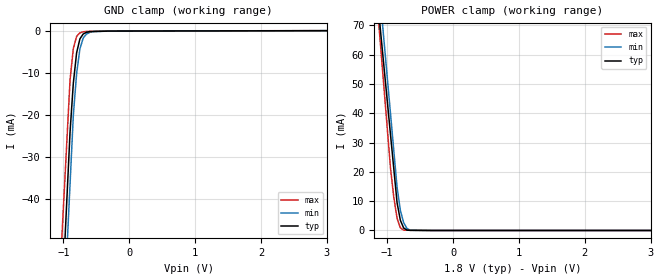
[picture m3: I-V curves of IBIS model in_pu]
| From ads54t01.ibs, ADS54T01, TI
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[Model] in_pu
Model_type Input
Vinl = 540.000mV
Vinh = 1.26000V
C_comp 746.000fF 715.000fF 777.000fF
| variable typ   min   max
[Voltage Range] 1.80000V 1.65000V 1.95000V
[POWER Clamp Reference] 1.80000V 1.65000V 1.95000V
[GND Clamp Reference] 0.00000V 0.00000V 0.00000V
[Temperature Range]   25   85   -40
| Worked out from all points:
|   GND clamp passes 1 mA (typ) near -0.71 V on its own axis
|   POWER clamp passes 1 mA (typ) near -0.75 V on its own axis
[GND Clamp]
-1.8V     -323.2mA   -332.7mA   -283mA
-900mV    -24.14mA   -36.54mA   -11.73mA
-850mV    -12.46mA   -20.09mA   -4.21mA
-800mV    -5.227mA   -10.16mA   -1.32mA
-750mV    -1.913mA   -4.295mA   -490.6uA
-700mV    -754.8uA   -1.715mA   -236.9uA
-650mV    -366.2uA   -786.3uA   -146uA
-550mV    -165.2uA   -183.1uA   -116uA
3.6V      48.02uA    56.76uA    57.43uA
[POWER Clamp]
-1.8V     230.9mA    253.7mA    256.7mA
-1.1V     67.72mA    77.61mA    62.82mA
-1.05V    56.06mA    65.03mA    48.96mA
-950mV    32.75mA    39.87mA    21.26mA
-900mV    21.1mA     27.29mA    11.36mA
-850mV    9.443mA    14.7mA     4.128mA
-800mV    3.464mA    6.824mA    873.1uA
-750mV    836.8uA    2.656mA    114.7uA
-700mV    156.5uA    667.8uA    101.9uA
-650mV    24.69uA    136.9uA    89.19uA
3.6V      0A         0A         0A
